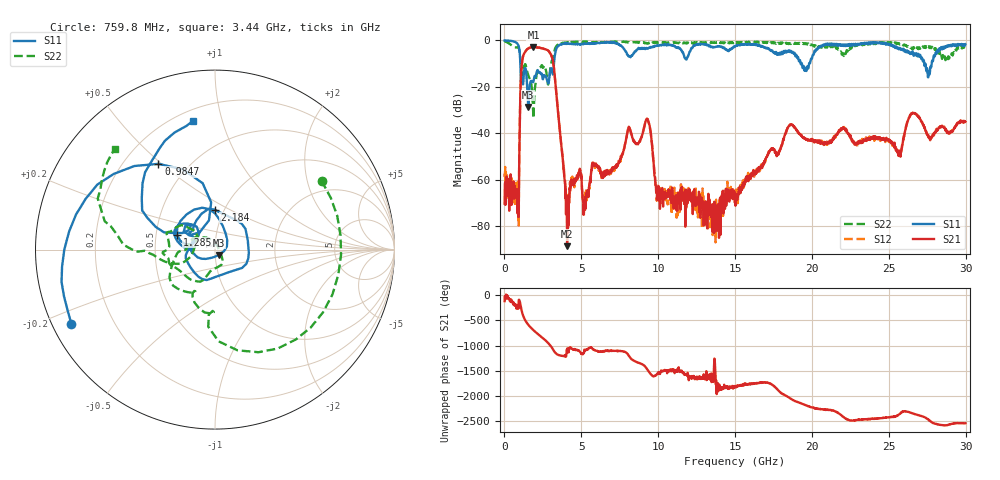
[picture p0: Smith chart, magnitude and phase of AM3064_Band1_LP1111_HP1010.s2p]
# Hz S DB R 50.0
!freq dBS11 angS11 dBS21 angS21 dBS12 angS12 dBS22 angS22
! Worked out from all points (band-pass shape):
!   1600 points, 10 MHz to 29.98 GHz, reference 50 ohm
!   highest |S21| = -2.85 dB at 1.884 GHz (marker M1); lowest = -88.7 dB at 4.077 GHz (marker M2)
!   |S21| within 3 dB of the highest: 1.266 GHz to 3 GHz (1.734 GHz wide, 81.3 % of centre)
!   lowest |S11| = -28.7 dB at 1.547 GHz (marker M3), VSWR 1.08, Z = 52.2 - j3.06 ohm
!   |S11| at or under -10 dB: 1.031 GHz to 3.221 GHz (2.19 GHz wide, 103 % of centre); 19.34 GHz to 19.82 GHz (472.7 MHz wide, 2.41 % of centre); 27.38 GHz to 27.79 GHz (415.5 MHz wide, 1.51 % of centre)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
!   |S22| runs from -33.6 to -0.2 dB; largest |S21 - S12| = 0.0099
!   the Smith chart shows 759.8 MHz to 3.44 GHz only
!   S11 on the Smith chart (normalised r, x): 759.8 MHz: 0.06, -0.24; 984.7 MHz: 0.34, +0.49; 1.285 GHz: 0.64, +0.11; 2.184 GHz: 0.90, +0.42; 3.44 GHz: 0.26, +0.81
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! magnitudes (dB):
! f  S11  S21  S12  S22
! 10 MHz  0.0  -70.4  -57.4  -0.2
! 759.8 MHz  -0.9  -67.1  -66.1  -3.0
! 984.7 MHz  -4.8  -40.9  -40.8  -4.8
! 1.285 GHz  -12.9  -5.6  -5.6  -11.0
! 1.547 GHz  -28.7  -3.5  -3.4  -14.9
! 1.884 GHz  -17.7  -2.8  -2.9  -33.6
! 2.184 GHz  -13.0  -3.1  -3.1  -13.2
! 3.046 GHz  -12.0  -6.5  -6.4  -9.7
! 3.44 GHz  -2.8  -27.7  -27.5  -2.0
! 4.077 GHz  -1.5  -88.7  -78.5  -0.8
! 5.015 GHz  -1.5  -58.4  -60.7  -0.6
! 9.288 GHz  -3.5  -33.9  -34.0  -1.3
! 10 GHz  -2.2  -65.5  -66.3  -0.9
! 13.81 GHz  -2.7  -79.1  -80.1  -0.9
! 15 GHz  -2.7  -65.7  -65.4  -1.2
! 18.57 GHz  -5.0  -36.4  -36.4  -1.2
! 19.99 GHz  -7.9  -42.8  -43.2  -1.8
! 25 GHz  -1.4  -42.8  -43.8  -1.1
! 25.71 GHz  -3.2  -49.7  -49.1  -1.8
! 26.59 GHz  -5.8  -31.4  -31.3  -3.2
! 27.56 GHz  -15.9  -40.8  -41.8  -2.6
! 29.98 GHz  -1.7  -35.0  -34.9  -2.9
